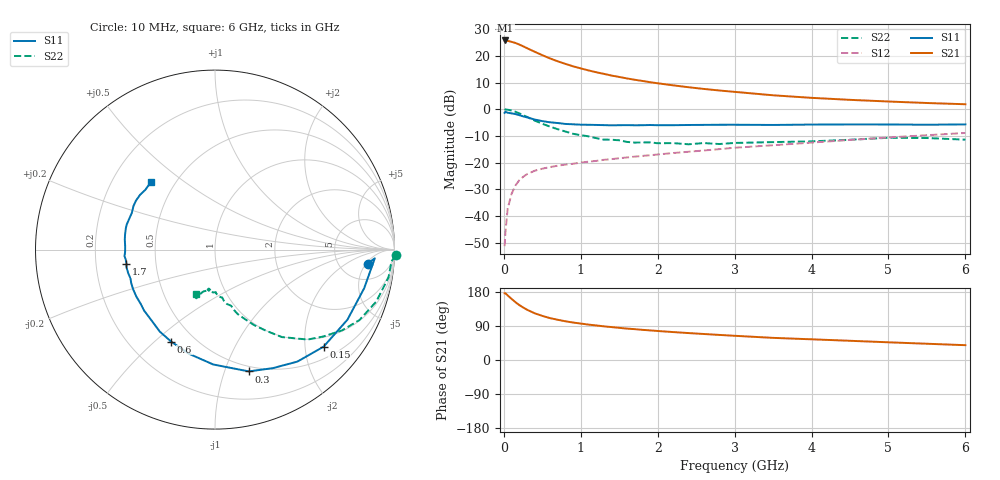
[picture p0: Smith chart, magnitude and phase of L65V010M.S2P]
!  INFINEON TECHNOLOGIES Small Signal Semiconductors
! BFR380L3 , Si-NPN RF-Transistor in TSLP-3-1
!  Vce=5 V,  Ic=10 mA
! Common Emitter S-Parameters:  07. March 2005
#  GHz  S  MA  R  50
! f  S11  S21  S12  S22
! GHz  Mag  Ang  Mag  Ang  Mag  Ang  Mag  Ang
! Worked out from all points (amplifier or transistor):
!   36 points, 10 MHz to 6 GHz, reference 50 ohm
!   highest |S21| = 25.8 dB at 20 MHz (marker M1)
!   |S21| within 3 dB of that: start of sweep to 309 MHz
!   unconditionally stable (mu >= 1): 2.487 GHz to 4.651 GHz
!   at 250 MHz: K = 0.22, MSG = 24.5 dB, |S12| = -25.4 dB
!   at 1.4 GHz: K = 0.83, MSG = 15.7 dB, |S12| = -18.7 dB
!   at 6 GHz: K = 0.95, MSG = 5.4 dB, |S12| = -8.9 dB
!   S11 on the Smith chart (normalised r, x): 10 MHz: 10, -6; 150 MHz: 0.76, -2.41; 300 MHz: 0.45, -1.21; 600 MHz: 0.37, -0.57; 1.7 GHz: 0.34, -0.07; 6 GHz: 0.37, +0.38
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0.01  0.8547 -5.2  19.42 176.1  0.0027 81.6  1.008 -1.8
0.02  0.8917 -3.1  19.46 176.2  0.0048 93.5  0.9856 -3.8
0.05  0.8586 -14.5  19.12 170.3  0.0137 82.6  0.9791 -9.1
0.1  0.8348 -27.9  18.34 161.4  0.0258 76.9  0.9443 -17.8
0.15  0.8115 -41.8  17.49 152.7  0.0369 69.9  0.8955 -26.0
0.2  0.7745 -53.7  16.33 145.1  0.0464 65.3  0.8383 -32.5
0.25  0.7346 -64.1  15.15 138.7  0.0538 60.3  0.7731 -38.8
0.3  0.7042 -74.5  13.97 132.8  0.0604 57.2  0.7202 -44.1
0.4  0.6401 -90.9  11.97 123.4  0.0701 52.1  0.6134 -52.6
0.5  0.598 -104.1  10.31 116.4  0.0766 49.5  0.5333 -57.9
0.6  0.5678 -115.5  8.952 110.5  0.0822 47.9  0.4715 -62.8
0.8  0.5293 -132.2  7.079 102.2  0.0916 46.9  0.3812 -70.6
0.9  0.5211 -139.3  6.375 98.9  0.0948 46.9  0.3454 -73.1
1.1  0.5104 -149.2  5.343 93.4  0.1037 48.1  0.3103 -77.6
1.4  0.4975 -161.2  4.277 86.9  0.1157 50.1  0.268 -82.7
1.7  0.4996 -170.9  3.572 81.4  0.1289 52.2  0.2369 -88.9
2.2  0.5011 177.6  2.805 73.7  0.1507 54.9  0.2315 -94.3
2.8  0.5108 166.4  2.244 66.2  0.1782 57.6  0.2223 -101.8
3.5  0.5066 156.2  1.824 58.4  0.2109 58.4  0.2416 -105.4
4.5  0.518 148.3  1.498 50.7  0.2652 59.9  0.2674 -109.0
5.5  0.5114 139.3  1.307 42.9  0.3254 58.6  0.2881 -111.7
6  0.5191 133.5  1.239 39.1  0.3584 57.3  0.2682 -112.9
